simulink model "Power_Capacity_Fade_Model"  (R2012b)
settings: Solver=ode4  StartTime=0.0  StopTime=300  FixedStep=0.001  RelTol=1e-3
undefined symbols (not defined in the file or in its folder): InitialSOC

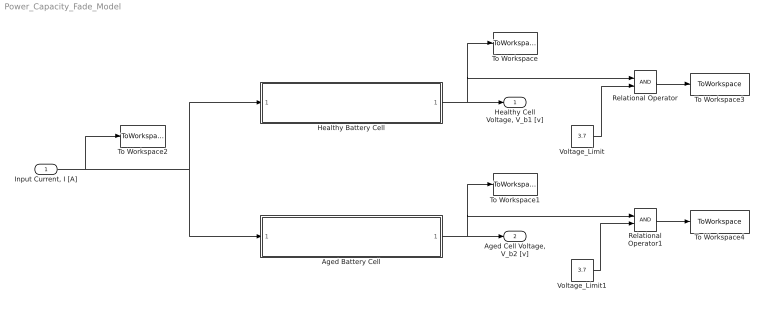
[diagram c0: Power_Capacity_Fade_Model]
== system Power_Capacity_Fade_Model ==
  "Input Current, I [A]" : Inport
  Aged Battery Cell : Subsystem
  Healthy Battery Cell : Subsystem
  Relational Operator : RelationalOperator  OutDataTypeStr=boolean
  Relational Operator1 : RelationalOperator  OutDataTypeStr=boolean
  To Workspace : ToWorkspace  VariableName=V_healthy  SampleTime=-1  SaveFormat=Structure With Time
  To Workspace1 : ToWorkspace  VariableName=V_aged  SampleTime=-1  SaveFormat=Structure With Time
  To Workspace2 : ToWorkspace  VariableName=InputCurrent  SampleTime=-1  SaveFormat=Structure With Time
  To Workspace3 : ToWorkspace  VariableName=Error_healthy  SampleTime=-1  SaveFormat=Structure With Time
  To Workspace4 : ToWorkspace  VariableName=Error_aged  SampleTime=-1  SaveFormat=Structure With Time
  Voltage_Limit : Constant  Value=3.7
  Voltage_Limit1 : Constant  Value=3.7
  "Healthy Cell Voltage, V_b1 [v]" : Outport
  "Aged Cell Voltage, V_b2 [v]" : Outport  Port=2
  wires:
  "Input Current, I [A]"/1 -> To Workspace2/1, Aged Battery Cell/1("InputCurrent, I_b [A]"), Healthy Battery Cell/1("InputCurrent, I_b [A]")
  Healthy Battery Cell/1("OutputVoltage, V_b [v]") -> To Workspace/1, Relational Operator/1, "Healthy Cell Voltage, V_b1 [v]"/1
  Aged Battery Cell/1("OutputVoltage, V_b [v]") -> To Workspace1/1, Relational Operator1/1, "Aged Cell Voltage, V_b2 [v]"/1
  Relational Operator1/1 -> To Workspace4/1
  Voltage_Limit/1 -> Relational Operator/2
  Voltage_Limit1/1 -> Relational Operator1/2
  Relational Operator/1 -> To Workspace3/1

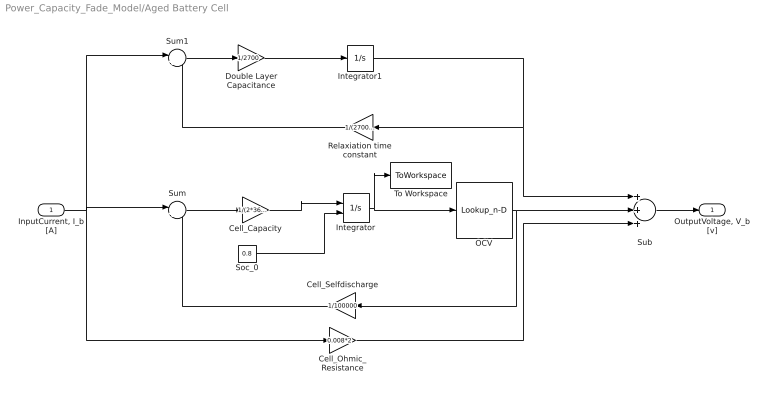
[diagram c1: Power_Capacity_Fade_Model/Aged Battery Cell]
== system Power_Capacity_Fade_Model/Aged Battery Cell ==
  "InputCurrent, I_b [A]" : Inport
  Cell_Capacity : Gain  Gain=1/(2*3600*0.8)
  Cell_Ohmic_Resistance : Gain  Gain=0.008*2
  Cell_Selfdischarge : Gain  Gain=1/100000
  Double Layer Capacitance : Gain  Gain=1/2700
  Integrator : Integrator  InitialConditionSource=external  InitialCondition=InitialSOC
  Integrator1 : Integrator
  OCV : Lookup_n-D  NumberOfTableDimensions=1  BreakpointsForDimension1=[0 0.1 0.2 0.3 0.4 0.5 0.6 0.7 0.8 0.9 1]  Table=[2.25 3.2 3.25 3.25 3.3 3.3 3.3 3.35 3.35 3.35 3.75]  RndMeth=Simplest
  Relaxiation time constant : Gain  Gain=1/(2700*0.011)
  Soc_0 : Constant  Value=0.8
  Sub : Sum  Inputs=+++
  Sum : Sum  Inputs=|+-
  Sum1 : Sum  Inputs=|+-
  To Workspace : ToWorkspace  VariableName=SOC_aged  SampleTime=-1  SaveFormat=Structure With Time
  "OutputVoltage, V_b [v]" : Outport
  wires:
  Soc_0/1 -> Integrator/2
  Sum1/1 -> Double Layer Capacitance/1
  Double Layer Capacitance/1 -> Integrator1/1
  Sum/1 -> Cell_Capacity/1
  Sub/1 -> "OutputVoltage, V_b [v]"/1
  Cell_Ohmic_Resistance/1 -> Sub/3
  Relaxiation time constant/1 -> Sum1/2
  Integrator1/1 -> Sub/1, Relaxiation time constant/1
  Cell_Selfdischarge/1 -> Sum/2
  Cell_Capacity/1 -> Integrator/1
  "InputCurrent, I_b [A]"/1 -> Sum/1, Cell_Ohmic_Resistance/1, Sum1/1
  OCV/1 -> Sub/2, Cell_Selfdischarge/1
  Integrator/1 -> To Workspace/1, OCV/1

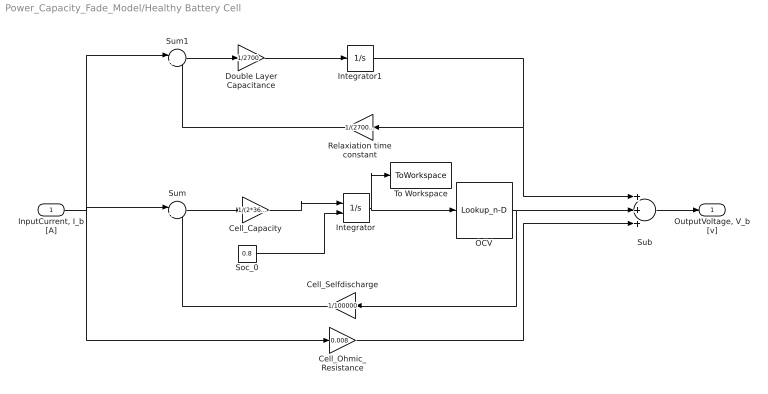
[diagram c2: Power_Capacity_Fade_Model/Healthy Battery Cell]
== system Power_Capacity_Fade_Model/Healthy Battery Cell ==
  "InputCurrent, I_b [A]" : Inport
  Cell_Capacity : Gain  Gain=1/(2*3600)
  Cell_Ohmic_Resistance : Gain  Gain=0.008
  Cell_Selfdischarge : Gain  Gain=1/100000
  Double Layer Capacitance : Gain  Gain=1/2700
  Integrator : Integrator  InitialConditionSource=external  InitialCondition=InitialSOC
  Integrator1 : Integrator
  OCV : Lookup_n-D  NumberOfTableDimensions=1  BreakpointsForDimension1=[0 0.1 0.2 0.3 0.4 0.5 0.6 0.7 0.8 0.9 1]  Table=[2.25 3.2 3.25 3.25 3.3 3.3 3.3 3.35 3.35 3.35 3.75]  RndMeth=Simplest
  Relaxiation time constant : Gain  Gain=1/(2700*0.011)
  Soc_0 : Constant  Value=0.8
  Sub : Sum  Inputs=+++
  Sum : Sum  Inputs=|+-
  Sum1 : Sum  Inputs=|+-
  To Workspace : ToWorkspace  VariableName=SOC_healthy  SampleTime=-1  SaveFormat=Structure With Time
  "OutputVoltage, V_b [v]" : Outport
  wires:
  Integrator/1 -> OCV/1, To Workspace/1
  OCV/1 -> Cell_Selfdischarge/1, Sub/2
  "InputCurrent, I_b [A]"/1 -> Sum1/1, Cell_Ohmic_Resistance/1, Sum/1
  Cell_Capacity/1 -> Integrator/1
  Cell_Selfdischarge/1 -> Sum/2
  Integrator1/1 -> Relaxiation time constant/1, Sub/1
  Relaxiation time constant/1 -> Sum1/2
  Cell_Ohmic_Resistance/1 -> Sub/3
  Sub/1 -> "OutputVoltage, V_b [v]"/1
  Sum/1 -> Cell_Capacity/1
  Double Layer Capacitance/1 -> Integrator1/1
  Sum1/1 -> Double Layer Capacitance/1
  Soc_0/1 -> Integrator/2
